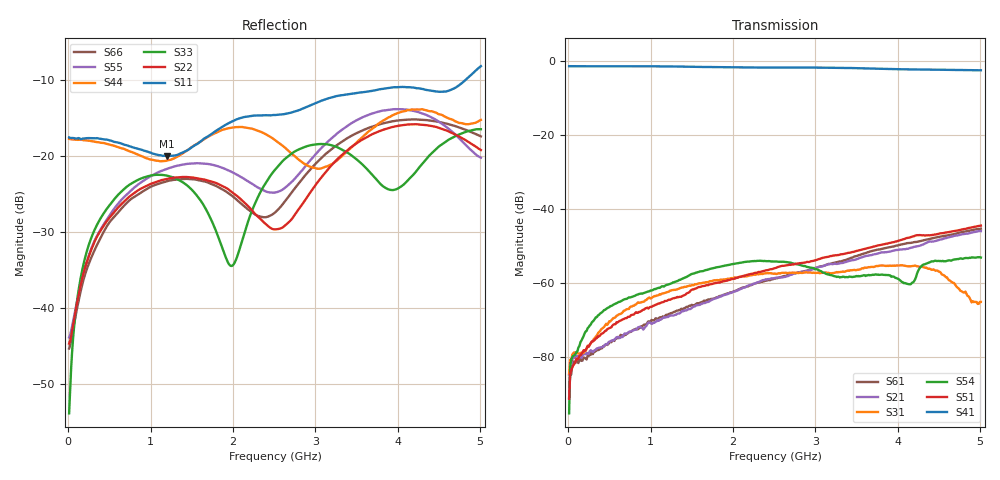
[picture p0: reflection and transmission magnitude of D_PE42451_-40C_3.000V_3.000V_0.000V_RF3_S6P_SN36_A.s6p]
! Device ID: PE42451
! Serial: 36
! Insertion: A
! Temp: -40C
! VDD: 3.000
! Control_Hi: 100.000
! Control_Lo: 0.000
! Logic State: RF3
! Port 1: RFC
! Port 2: RF1
! Port 3: RF2
! Port 4: RF3
! Port 5: RF4
! Port 6: RF5
! V1 = 3.00
! V2 = 3.00
! V3 = 0.00
! V4 = 0.00
! IDD: 1.323290e-05
#  Hz  S  RI  R  50
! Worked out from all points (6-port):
!   401 points, 10 MHz to 5.01 GHz, reference 50 ohm
!   strongest paths, dB at 10 MHz, 1.26 GHz, 2.51 GHz, 3.76 GHz, 5.01 GHz:
!     S41: -1.3, -1.4, -1.7, -2.0, -2.4
!     S51: -91.5, -64.3, -56.1, -49.9, -44.5
!     S54: -95.4, -60.1, -54.2, -57.8, -53.2
!     S31: -84.6, -62.0, -57.5, -55.5, -65.2
!     S21: -84.9, -68.9, -58.7, -52.1, -46.0
!     S61: -91.2, -68.2, -58.9, -51.0, -45.3
!   lowest |S11| = -20.0 dB at 1.198 GHz (marker M1), VSWR 1.22, Z = 55.6 - j8.94 ohm
!   |S11| at or under -10 dB: start of sweep to 4.828 GHz
